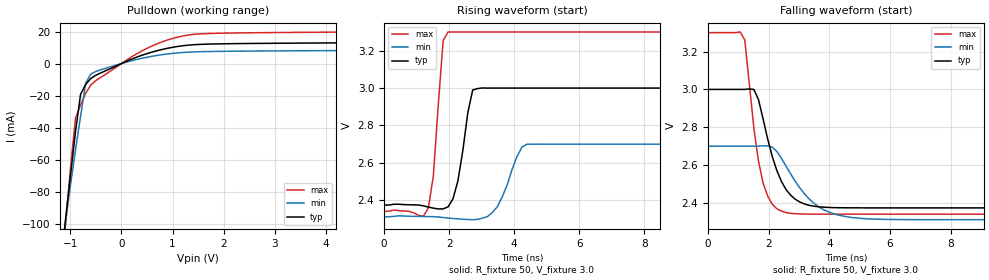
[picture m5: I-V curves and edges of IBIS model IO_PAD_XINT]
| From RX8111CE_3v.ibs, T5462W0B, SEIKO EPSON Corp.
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[Model]   IO_PAD_XINT
Model_type Open_drain
Enable Active-High
Polarity Non-Inverting
Vmeas=1.50
Vref=3.3
Rref=5000
C_comp   2.5p   2.0p   3.0p
[Temperature Range] 25   105   -40
[Voltage Range]   3.0   2.7   3.3
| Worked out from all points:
|   slope of the pulldown table from 0 to 0.45 V, typ, clamps not added: 79 ohm
|   falling waveform, R_fixture 50, V_fixture 3.0: 20-80 % time 702ps typ, 1.1ns min, 470ps max; typ from 3 V to 2.37 V
|   rising waveform, R_fixture 50, V_fixture 3.0: 20-80 % time 320ps typ, 511ps min, 238ps max; typ from 2.37 V to 3 V
[Pulldown]
-3V       -702.1mA   -577.4mA   -866.5mA
-1.1V     -99.04mA   -100.3mA   -102.6mA
-900mV    -42.59mA   -53.98mA   -34.23mA
-800mV    -19.2mA    -32.95mA   -25.77mA
-700mV    -13.01mA   -12.25mA   -18.5mA
-600mV    -9.326mA   -6.551mA   -13.4mA
-500mV    -7.242mA   -4.883mA   -10.62mA
500mV     6.223mA    3.955mA    9.514mA
900mV     9.547mA    6.005mA    14.7mA
1.3V      11.49mA    7.126mA    17.8mA
5V        13.19mA    8.301mA    20.03mA
6V        14.3mA     9.054mA    21.64mA
[Falling Waveform]
R_fixture=50
V_fixture=3.0
V_fixture_min=2.7
V_fixture_max=3.3
0s        3V         2.7V       3.3V
1.212ns   3V         2.7V       3.262V
1.515ns   3V         2.7V       2.792V
1.818ns   2.843V     2.702V     2.505V
2.121ns   2.645V     2.695V     2.393V
2.424ns   2.513V     2.635V     2.357V
2.879ns   2.42V      2.514V     2.343V
3.485ns   2.383V     2.4V       2.341V
4.697ns   2.375V     2.324V     2.341V
15ns      2.374V     2.312V     2.341V
[Rising Waveform]
R_fixture=50
V_fixture=3.0
V_fixture_min=2.7
V_fixture_max=3.3
0s        2.374V     2.312V     2.341V
1.364ns   2.364V     2.313V     2.359V
1.515ns   2.358V     2.312V     2.528V
1.818ns   2.354V     2.308V     3.254V
1.97ns    2.365V     2.305V     3.3V
2.273ns   2.504V     2.301V     3.3V
2.727ns   2.99V      2.296V     3.3V
2.879ns   2.997V     2.298V     3.3V
4.394ns   3V         2.7V       3.3V
15ns      3V         2.7V       3.3V
[Ramp]
R_load=50
dV/dt_r   3.755E-1/3.145E-10   2.329E-1/5.015E-10   5.754E-1/2.252E-10
dV/dt_f   3.755E-1/6.971E-10   2.329E-1/1.094E-9   5.754E-1/4.581E-10
|[End   IO_PAD_XINT
